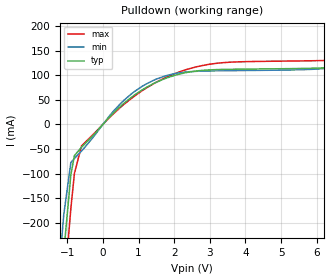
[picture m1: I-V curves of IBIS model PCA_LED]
| Philips Semiconductors Inc.
| Specialty Logic Products -- Albuquerque, NM
| IBIS model of PCA9553
| 4-bit I2C LED driver with programmable blink rates
| SO 8-pin Package
| TSSOP 8-pin Package
[IBIS Ver]   2.1
[Comment Char]   |_char
[File name]   pca9553.ibs
[File Rev]   1.0
[Date]   Apr 22, 2002
[Source]
Generated from ITK by TGA + GJ in ABQ
[Notes]
[Disclaimer]
Philips Semiconductors warrants and represents that the IBIS models
identified herein are owned by Philips Semiconductors (PHILIPS). The models
provided are not warranted as fully representing all of the operating
characteristics and specifications of the semiconductor products to which the
models relate. Moreover, unless there is a signed, written agreement to the
contrary, these models are furnished on an "as is" basis without support or
warranty of any kind, either expressed or implied, regarding the use thereof,
and PHILIPS specifically disclaims all implied warranties of merchantability and
fitness of the models for any purpose. PHILIPS does not assume any liability
arising out of the application or use of these SPICE models including
infringement of patents and copyrights, nor does PHILIPS convey any license
under its patents and copyrights or the rights of others. PHILIPS provides IBIS
models as a service to our customers. You and your company shall not distribute,
convey, sell, or give these models to anyone else without receiving prior
written permission from PHILIPS. PHILIPS reserves the right to make changes
without notice to these IBIS models to improve reliability, function, or
design.
[Copyright]
Copyright 2002, Philips Semiconductors, All rights reserved.
[Component]   PCA9553-1D
[Manufacturer]   Philips Semiconductors
| [Package]   SO8
[Package]
|   typ   min   max
R_pkg   4.81E-02  4.14E-02  5.47E-02
L_pkg   1.88E-09  1.54E-09  2.21E-09
C_pkg   4.49E-13  4.17E-13  4.81E-13
[Pin] signal_name   model_name   R_pin   L_pin   C_pin
1   LED0   PCA_LED   5.47E-02 2.21E-09  4.81E-13
2   LED1   PCA_LED   4.14E-02 1.54E-09  4.20E-13
3   LED2   PCA_LED   4.14E-02 1.55E-09  4.20E-13
4   VSS   GND   5.47E-02 2.21E-09  4.80E-13
5   LED3   PCA_LED   5.47E-02 2.21E-09  4.78E-13
6   SCL   PCA_IN   4.14E-02 1.55E-09  4.17E-13
7   SDA   PCA_IN   4.14E-02 1.54E-09  4.17E-13
8   VDD   POWER   5.47E-02 2.21E-09  4.79E-13
[Component]   PCA9553-1DP
[Manufacturer]   Philips Semiconductors
| [Package]   TSSOP8
[Package]
|   typ   min   max
R_pkg   33.7m   30.1m   37.3m
L_pkg   1.74nH   1.67nH   1.81nH
C_pkg   0.428pF   0.422pF   0.434pF
[Pin] signal_name   model_name   R_pin   L_pin   C_pin
1   LED0   PCA_LED   37.3m   1.81nH   0.428pF
2   LED1   PCA_LED   30.1m   1.67nH   0.422pF
3   LED2   PCA_LED   30.1m   1.67nH   0.428pF
4   VSS   GND   37.3m   1.81nH   0.434pF
5   LED3   PCA_LED   37.3m   1.81nH   0.428pF
6   SCL   PCA_IN   30.1m   1.67nH   0.422pF
7   SDA   PCA_IN   30.1m   1.67nH   0.428pF
8   VDD   POWER   37.3m   1.81nH   0.434pF
[Model]   PCA_IN
Model_type Input
Vinh=4.5
Vinl=0
C_comp   0.5p   0.5p   0.5p
[Temperature Range] 25   -40   85
[Voltage Range]   5   4.5   5.5
[Pullup Reference]  5   4.5   5.5
[Pulldown Reference]0   0   0
[POWER Clamp Reference]5   4.5   5.5
[GND Clamp Reference]0   0   0
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| Models and submodels in the file (2): PCA_IN (Input), PCA_LED (Open_drain)
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[Model]   PCA_LED
Model_type Open_drain
C_comp   0.5p   0.5p   0.5p
[Temperature Range] 25   -40   85
[Voltage Range]   5   4.5   5.5
[Pullup Reference]  5   4.5   5.5
[Pulldown Reference]0   0   0
[POWER Clamp Reference]5   4.5   5.5
[GND Clamp Reference]0   0   0
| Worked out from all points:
|   slope of the pulldown table from 0 to 0.75 V, typ, clamps not added: 14.4 ohm
[Pulldown]
-5V       -4.084A    -4.011A    -4.161A
-1.2V     -351.6mA   -271.8mA   -435.1mA
-1.1V     -261.3mA   -184.3mA   -343.6mA
-900mV    -102.8mA   -77.38mA   -171.4mA
-800mV    -63.48mA   -69.33mA   -99.77mA
-600mV    -46.52mA   -54.11mA   -43.74mA
500mV     37.17mA    42.63mA    34.94mA
1.5V      85.61mA    91.93mA    85.69mA
3.2V      111.3mA    108.8mA    124.2mA
7.1V      119.9mA    120.6mA    133mA
8.6V      143.3mA    149.6mA    152.1mA
10V       186mA      197.9mA    192mA
[Ramp]
R_load=250
dV/dt_r   2.858E+0/9.272E-10   2.878E+0/8.595E-10   2.857E+0/9.994E-10
dV/dt_f   2.675E+0/9.656E-9   2.600E+0/1.045E-8   2.713E+0/8.615E-9
